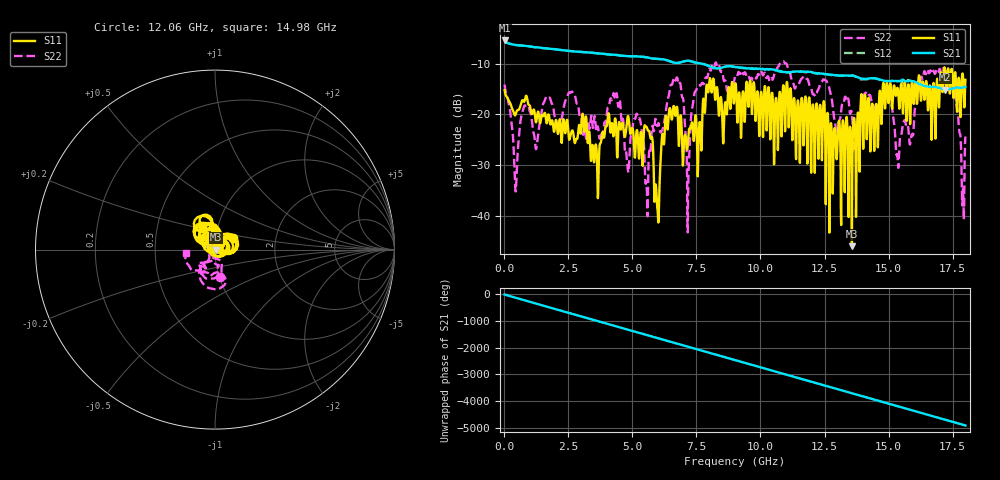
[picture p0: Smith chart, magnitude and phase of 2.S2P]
!Agilent Technologies,E5071C,MY46316741,A.11.02
!Date: Thu Sep 29 15:37:53 2022
!Data & Calibration Information:
!Freq	S11:SOLT2(ON)	S21:SOLT2(ON)	S12:SOLT2(ON)	S22:SOLT2(ON)
!PortZ  Port1:50+j0  Port2:50+j0
!Above PortZ is port z conversion or system Z0 setting when saving the data.
!When reading, reference impedance value at option line is always used.
# Hz S dB R 50
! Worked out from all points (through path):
!   1800 points, 10 MHz to 18 GHz, reference 50 ohm
!   highest |S21| = -5.39 dB at 10 MHz (marker M1); lowest = -15.1 dB at 17.19 GHz (marker M2)
!   group delay of S21, straight-line fit = 758 ps
!   lowest |S11| = -46.0 dB at 13.57 GHz (marker M3), VSWR 1.01, Z = 50.5 + j0.0273 ohm
!   |S11| at or under -10 dB: start of sweep to end of sweep
!   |S22| runs from -43.3 to -9.5 dB; largest |S21 - S12| = 0.022
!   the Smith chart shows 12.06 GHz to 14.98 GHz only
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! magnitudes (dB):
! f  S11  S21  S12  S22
! 10 MHz  -15.2  -5.4  -5.4  -14.1
! 450 MHz  -19.8  -6.3  -6.3  -35.0
! 830 MHz  -16.5  -6.5  -6.5  -18.3
! 3.01 GHz  -22.2  -7.7  -7.7  -21.0
! 3.59 GHz  -26.4  -7.9  -7.9  -23.4
! 4.33 GHz  -20.8  -8.2  -8.2  -17.0
! 4.79 GHz  -21.2  -8.5  -8.5  -29.4
! 5.25 GHz  -28.4  -8.6  -8.5  -20.9
! 5.56 GHz  -22.5  -8.7  -8.7  -34.3
! 6.01 GHz  -41.4  -9.0  -9.0  -21.7
! 6.52 GHz  -20.6  -9.6  -9.6  -14.1
! 6.92 GHz  -22.4  -9.7  -9.6  -16.0
! 7.16 GHz  -25.9  -9.4  -9.4  -43.3
! 7.51 GHz  -23.2  -9.8  -9.9  -15.0
! 7.97 GHz  -15.4  -10.4  -10.4  -11.6
! 9.01 GHz  -14.1  -10.6  -10.7  -12.5
! 12.01 GHz  -21.0  -11.7  -11.7  -15.5
! 13.57 GHz  -46.0  -12.3  -12.3  -20.0
! 15.01 GHz  -17.3  -13.4  -13.4  -15.9
! 15.36 GHz  -14.9  -13.4  -13.4  -29.2
! 17.19 GHz  -10.8  -15.1  -15.1  -11.8
! 18 GHz  -13.2  -14.6  -14.7  -24.4
